(* Logix 5000 AddOnInstructionDefinition export AV6A; software revision 20.01 *)

ADD_ON_INSTRUCTION AV6A   (* revision 1.0 *)
// Ethernet IP Control Block For AV6A Multi-turn Absolute Encoder
// Help:
// THIS AOI WILL SCALE THE POSITION TO ENGINEERING UNITS USING THE "Pulse_Per_Unit" INPUT
// "Raw_Cnts_Out" WILL SHOW THE ENCODER RAW COUNT VALUE
// THE SPEED FEEDBACK OUTPUT WILL BE IN SCALED TO RPM's
VAR_INPUT
   Raw_Counts : DINT; {access Read Only, required}   // Encoder Raw Counts
   Raw_Speed : DINT; {access Read Only, required}   // Encoder Raw Speed
   Conn_Flt : BOOL; {access Read Only, required}   // Encoder Connection Faulted Raw Input
   Pulse_Per_Rev : DINT; {access Read Only, required}   // Encoder Pulses Per Revolution
   Pulse_Per_Unit : REAL; {access Read Only, required}   // Pulses / Unit
   Unit_Max_Range : REAL; {access Read Only, required}   // The Maximum Allowable Scaled Units Before Faulting
   Motor_Spd_Fdbk : REAL; {access Read Only, required}   // Motor Speed Feedback Used For Direction Fault Detection
   Dir_Chk_Spd : REAL; {access Read Only, required}   // Diection Check Speed Minimum In Percent
END_VAR
VAR_OUTPUT
   Pos_Fdbk : REAL; {access Read Only, required}   // Position Feedback in Units
   Spd_Fdbk : REAL; {access Read Only, required}   // Speed Feedback In Units Per Minute
   Comm_Loss : BOOL; {access Read Only, required}   // Encoder Communication Loss
   Out_Of_Range : BOOL; {access Read Only, required}   // Encoder Is Out Of Range
   Dir_Flt : BOOL; {access Read Only, required}   // Encoder Wrong Direction Fault
   Spd_Fdbk_RPM : REAL; {access Read Only}   // Encoder Speed Feedback In RPM's
END_VAR
VAR
   temp : REAL; {access None}
   Conn_Flt_Tmr : TIMER := (PRE := 100); {access None}
   Dir_Flt_Tmr : TIMER := (PRE := 500); {access None}
   Neg_Dir_Chk_Spd : REAL; {access None}
END_VAR

ROUTINE Logic   (* ladder *)
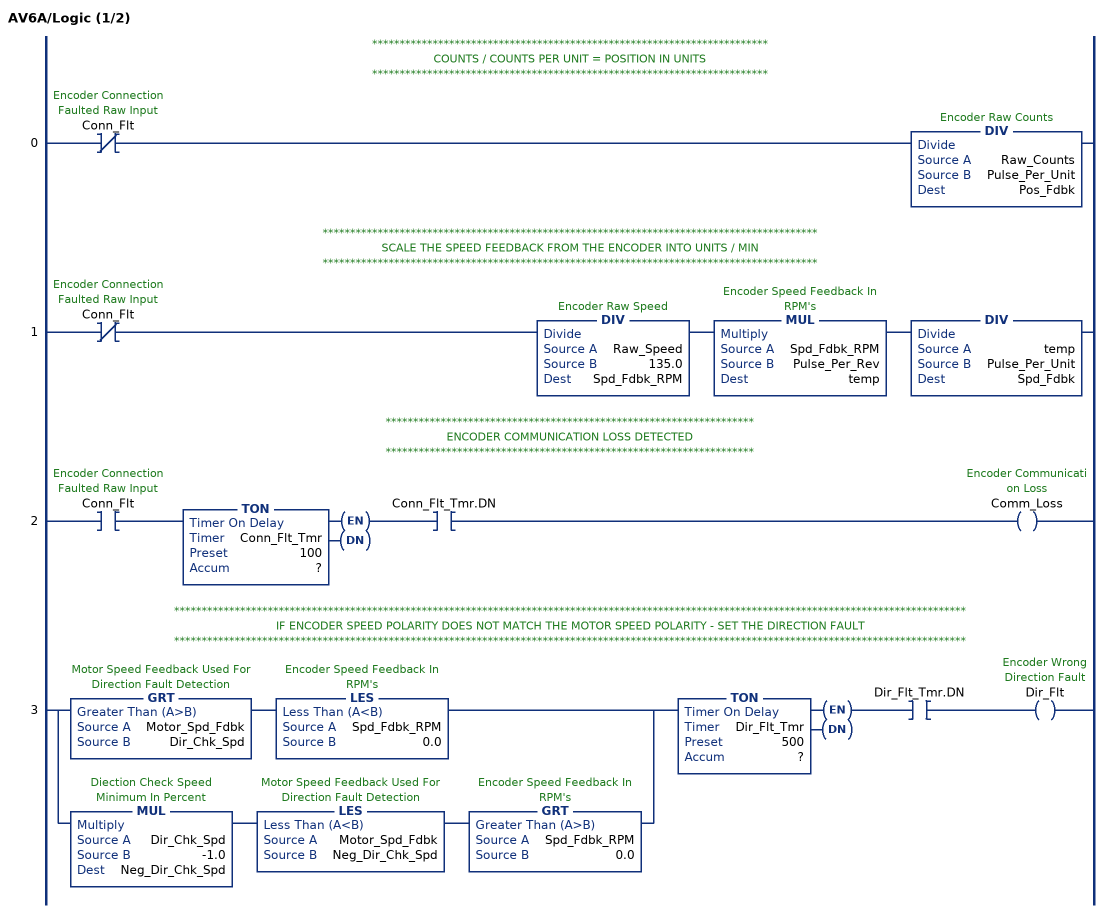
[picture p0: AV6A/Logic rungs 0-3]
   // ************************************************************************
   // COUNTS / COUNTS PER UNIT = POSITION IN UNITS
   // ************************************************************************
   0: XIO(Conn_Flt)DIV(Raw_Counts,Pulse_Per_Unit,Pos_Fdbk);
   // ******************************************************************************************
   // SCALE THE SPEED FEEDBACK FROM THE ENCODER INTO UNITS / MIN
   // ******************************************************************************************
   1: XIO(Conn_Flt)DIV(Raw_Speed,135.0,Spd_Fdbk_RPM)MUL(Spd_Fdbk_RPM,Pulse_Per_Rev,temp)DIV(temp,Pulse_Per_Unit,Spd_Fdbk);
   // *******************************************************************
   // ENCODER COMMUNICATION LOSS DETECTED
   // *******************************************************************
   2: XIC(Conn_Flt)TON(Conn_Flt_Tmr,?,?)XIC(Conn_Flt_Tmr.DN)OTE(Comm_Loss);
   // ************************************************************************************************************************************************
   // IF ENCODER SPEED POLARITY DOES NOT MATCH THE MOTOR SPEED POLARITY - SET THE DIRECTION FAULT
   // ************************************************************************************************************************************************
   3: [GRT(Motor_Spd_Fdbk,Dir_Chk_Spd) LES(Spd_Fdbk_RPM,0.0) ,MUL(Dir_Chk_Spd,-1.0,Neg_Dir_Chk_Spd) LES(Motor_Spd_Fdbk,Neg_Dir_Chk_Spd) GRT(Spd_Fdbk_RPM,0.0) ]TON(Dir_Flt_Tmr,?,?)XIC(Dir_Flt_Tmr.DN)OTE(Dir_Flt);
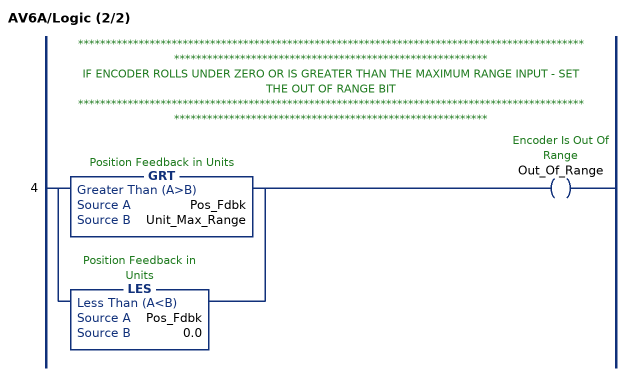
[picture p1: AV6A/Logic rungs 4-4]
   // *****************************************************************************************************************************************************
   // IF ENCODER ROLLS UNDER ZERO OR IS GREATER THAN THE MAXIMUM RANGE INPUT - SET THE OUT OF RANGE BIT
   // *****************************************************************************************************************************************************
   4: [GRT(Pos_Fdbk,Unit_Max_Range) ,LES(Pos_Fdbk,0.0) ]OTE(Out_Of_Range);
END_ROUTINE
END_ADD_ON_INSTRUCTION
